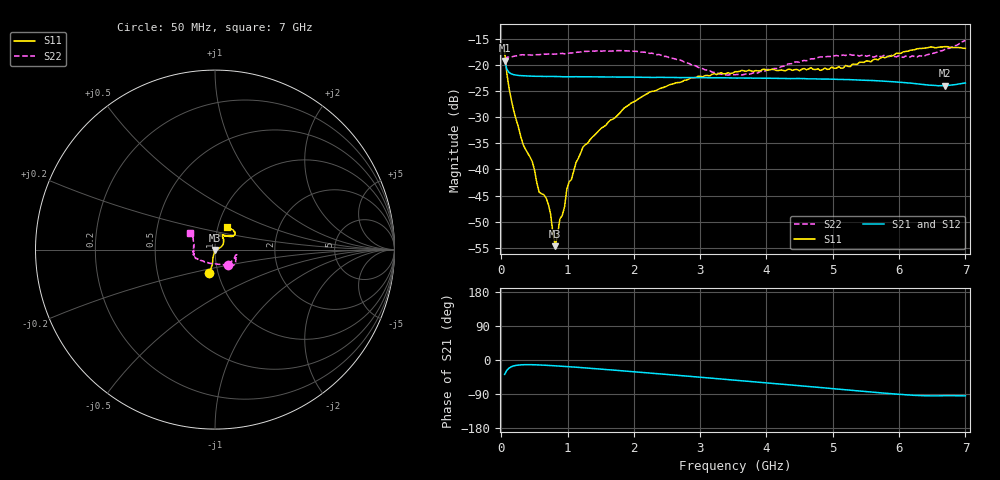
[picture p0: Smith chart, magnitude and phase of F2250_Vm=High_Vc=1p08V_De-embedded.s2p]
! Integrated Device Technology
! Corporate Headquarters
! 6024 Silver Creek Valley Road
! San Jose, CA 95138  USA
! Phone:  1-408-284-8200
! Toll Free:  1-800-223-1366
! Webpage:  http://www.idt.com/
! Timing and RF Division
! 515 Groton Road, Suite 102
! Westford, MA 01886-6024
! Device:  F2250
! Description: Voltage Variable RF Attenuator
! Frequency:  50.0 -  6000.00 MHz
! Package:  3x3 mm Thin QFN Plastic Package: 16 pin
! Ports:  2 RF, 3 DC
!  Pin  1  = GND
!  Pin  2  = NC
!  Pin  3  = RF1  = Port 1
!  Pin  4  = NC
!  Pin  5  = GND
!  Pin  6  = GND
!  Pin  7  = GND
!  Pin  8  = GND
!  Pin  9  = NC
!  Pin 10  = RF2  = Port 2
!  Pin 11  = NC
!  Pin 12  = GND
!  Pin 13  = GND
!  Pin 14  = VCNTRL
!  Pin 15  = VDD
!  Pin 16  = VMODE
! Vcntrl:  1.080 Volts
! Vmode:  +3.300 Volts
! Vdd:  +3.30  Volts
! Current:  1.330 mA
! Data:  The device was measured on a the F2250 evaluation board which has
!  individual transmission lines to the RF pins.  Data was collected
!  using a calibrated network analyzer.  The evaluation board was
!  de-embedded using a TRL calibration technique.
!  The reference plane is the edge of the package pin.
! Misc:  SN 10
!  Action Tracker AT0258
! Date Measured:  2014-11-26
! Date:  2015-10-15  MJV
! Note:
!  Integrated Device Technology supplies this data as a sample of measured
!  data at the package pin for this product.  Your particular data for this
!  product may vary.
!  Data was taken at 25 degrees C.
!  Integrated Device Technology reserves the right to change this data at anytime.
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# GHz S dB R 50
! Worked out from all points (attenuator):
!   201 points, 50 MHz to 7 GHz, reference 50 ohm
!   highest |S21| = -19.20 dB at 50 MHz (marker M1); lowest = -24.0 dB at 6.687 GHz (marker M2)
!   lowest |S11| = -54.7 dB at 814.5 MHz (marker M3), VSWR 1.00, Z = 50.1 - j0.13 ohm
!   |S11| at or under -10 dB: start of sweep to end of sweep
!   |S22| runs from -22.0 to -15.4 dB; largest |S21 - S12| = 0.00026
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0.05  -17.42 -103.7  -19.20 -38.1  -19.20 -38.0  -19.05 -48.3
0.1195  -24.67 -102.2  -21.52 -21.0  -21.51 -21.0  -18.54 -18.2
0.189  -28.86 -105.0  -21.91 -15.5  -21.91 -15.5  -18.39 -14.1
0.328  -35.21 -105.7  -22.11 -12.5  -22.11 -12.5  -18.10 -13.0
0.467  -38.49 -109.7  -22.19 -12.4  -22.18 -12.4  -18.17 -14.5
0.57125  -44.32 -102.8  -22.22 -13.0  -22.21 -13.1  -18.09 -16.9
0.71025  -46.68 -87.8  -22.25 -14.3  -22.23 -14.3  -17.96 -19.7
0.8145  -54.66 -44.7  -22.25 -15.4  -22.25 -15.4  -17.98 -22.1
0.884  -49.48 -22.7  -22.27 -16.1  -22.28 -16.1  -17.89 -24.2
0.9535  -47.18 -32.7  -22.30 -16.9  -22.28 -16.9  -17.92 -25.2
0.98825  -43.81 -22.4  -22.30 -17.3  -22.28 -17.3  -17.86 -25.9
1.2315  -35.75 6.1  -22.30 -20.4  -22.29 -20.4  -17.48 -30.4
1.857  -28.24 24.9  -22.37 -29.0  -22.39 -29.0  -17.33 -38.5
2.37825  -24.64 36.8  -22.41 -36.4  -22.43 -36.4  -18.05 -45.7
2.86475  -22.49 50.1  -22.46 -43.4  -22.46 -43.5  -20.01 -58.2
3.525  -21.33 67.1  -22.55 -53.1  -22.55 -53.2  -21.93 -97.8
4.7065  -20.90 69.7  -22.70 -71.0  -22.68 -71.1  -18.87 -153.4
5.15825  -20.64 53.5  -22.83 -78.0  -22.83 -78.0  -18.16 -161.9
5.85325  -18.30 38.2  -23.20 -88.5  -23.20 -88.6  -18.45 -176.1
6.3745  -16.83 39.3  -23.78 -94.4  -23.77 -94.5  -18.41 165.2
6.68725  -16.55 46.5  -24.03 -94.2  -24.03 -94.3  -17.10 151.2
7  -16.89 61.9  -23.49 -94.6  -23.51 -94.7  -15.37 146.4
